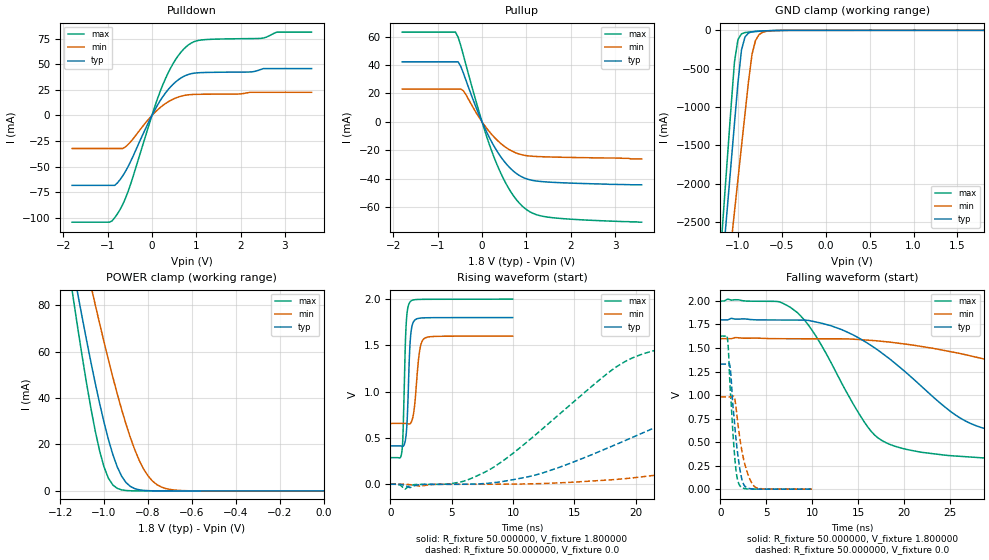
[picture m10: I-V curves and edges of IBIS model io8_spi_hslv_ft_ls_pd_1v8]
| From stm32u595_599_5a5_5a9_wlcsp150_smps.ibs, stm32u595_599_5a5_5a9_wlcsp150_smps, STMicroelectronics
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|   Model io8_spi_hslv_ft_ls_pd_1v8
[Model]  io8_spi_hslv_ft_ls_pd_1v8
Model_type I/O
Polarity   Non-Inverting
Enable   Active-Low
Vinl =   0.540000V
Vinh =   1.260000V
Vmeas =  0.900000V
Cref =   50.000000pF
Rref =   100.000000M
Vref =   0.0V
C_comp   3.338700pF   3.332500pF   3.379000pF
[Temperature Range]   25.000000   0.140000k   -40.000000
[Pullup Reference]   1.800000V   1.600000V   2.000000V
[Pulldown Reference]   0.0V   0.0V   0.0V
[POWER Clamp Reference]   1.800000V   1.600000V   2.000000V
[GND Clamp Reference]   0.0V   0.0V   0.0V
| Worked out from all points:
|   slope of the pulldown table from 0 to 0.27 V, typ, clamps not added: 13.6 ohm
|   slope of the pullup table from 0 to 0.27 V, typ, clamps not added: 15.9 ohm
|   GND clamp passes 1 mA (typ) near -0.50 V on its own axis
|   POWER clamp passes 1 mA (typ) near -0.86 V on its own axis
|   rising waveform, R_fixture 50.000000, V_fixture 1.800000: 20-80 % time 238ps typ, 381ps min, 212ps max; typ from 0.414 V to 1.8 V
|   rising waveform, R_fixture 50.000000, V_fixture 0.0: 20-80 % time 15.2ns typ, 31.7ns min, 8.92ns max; typ from 0 V to 1.33 V
|   falling waveform, R_fixture 50.000000, V_fixture 1.800000: 20-80 % time 10.9ns typ, 26.5ns min, 6.1ns max; typ from 1.8 V to 0.414 V
|   falling waveform, R_fixture 50.000000, V_fixture 0.0: 20-80 % time 792ps typ, 1.07ns min, 617ps max; typ from 1.33 V to 0 V
[Pulldown]
|Voltage   I(typ)   I(min)   I(max)
-1.8V     -68.38mA   -32.32mA   -104.4mA
-960mV    -68.38mA   -32.32mA   -104.4mA
-780mV    -66.07mA   -32.32mA   -96.42mA
-540mV    -50.22mA   -28.51mA   -74.66mA
0V        -10fA      -700fA     0A
240mV     18.04mA    9.598mA    29.41mA
480mV     30.68mA    16.02mA    50.95mA
780mV     39.47mA    19.98mA    67.56mA
1.14V     41.99mA    20.77mA    74.01mA
2.46V     45.09mA    22.69mA    75.44mA
2.82V     45.91mA    22.69mA    81.6mA
3.6V      45.91mA    22.69mA    81.6mA
[Pullup]
|Voltage   I(typ)   I(min)   I(max)
-1.8V     42.21mA    23.08mA    63.11mA
-600mV    42.21mA    23.08mA    63.11mA
-540mV    42.21mA    23.08mA    59.57mA
-420mV    34.21mA    21.83mA    46.75mA
0V        0A         0A         0A
300mV     -18.63mA   -11.6mA    -27.18mA
600mV     -31.41mA   -19.24mA   -46.67mA
780mV     -36.41mA   -22mA      -54.89mA
960mV     -39.54mA   -23.51mA   -60.64mA
1.2V      -41.44mA   -24.28mA   -64.93mA
1.56V     -42.42mA   -24.69mA   -67.24mA
3.6V      -44.2mA    -26mA      -70.5mA
[GND_clamp]
|Voltage   I(typ)   I(min)   I(max)
-1.8V     -9.908A    -9.683A    -9.994A
-1.2V     -3.383A    -4.084A    -2.934A
-1.16V    -2.841A    -3.655A    -2.294A
-1.12V    -2.299A    -3.226A    -1.656A
-1.04V    -1.218A    -2.369A    -414.2mA
-1V       -684.7mA   -1.941A    -119.2mA
-960mV    -257.2mA   -1.514A    -45.67mA
-920mV    -87.04mA   -1.089A    -28.94mA
-840mV    -19.36mA   -312.8mA   -18.98mA
-800mV    -13.56mA   -132.4mA   -15.51mA
-720mV    -8.053mA   -25.67mA   -9.504mA
1.8V      45.71uA    33.32uA    56.11uA
[POWER_clamp]
|Voltage   I(typ)   I(min)   I(max)
-1.8V     470.8mA    433.7mA    554.6mA
-1.14V    95.25mA    122.7mA    82.82mA
-1.12V    84.97mA    114mA      70.27mA
-1.06V    55.51mA    88.42mA    35.67mA
-1.04V    46.34mA    80.15mA    25.76mA
-1V       29.51mA    64.13mA    10.3mA
-940mV    10.39mA    41.86mA    1.109mA
-900mV    3.624mA    28.77mA    182.8uA
-840mV    490.7uA    13.24mA    11.35uA
-800mV    116.8uA    6.532mA    1.77uA
-740mV    13.2uA     1.724mA    109.3nA
0V        0A         18.75nA    0A
[Ramp]
| variable   typ   min   max
dV/dt_r  0.79740/15.22129n   0.58772/31.69284n   0.97632/8.91131n
dV/dt_f  0.83143/10.92816n   0.56537/26.52287n   1.02743/6.08253n
R_load = 50.000000
[Rising Waveform]
R_fixture= 50.000000
V_fixture= 1.800000
V_fixture_min= 1.600000
V_fixture_max= 2.000000
|time   V(typ)   V(min)   V(max)
0s        413.8mV    656.5mV    287.1mV
940.9ps   411.3mV    656.6mV    348mV
1.041ns   410.7mV    656.6mV    560.4mV
1.281ns   522.4mV    656.1mV    1.694V
1.401ns   766mV      654.2mV    1.883V
1.602ns   1.498V     653.4mV    1.967V
1.882ns   1.752V     752.7mV    1.99V
2.382ns   1.793V     1.432V     1.996V
2.763ns   1.797V     1.573V     1.997V
9.97ns    1.8V       1.599V     2V
[Rising Waveform]
R_fixture= 50.000000
V_fixture= 0.0
V_fixture_min= 0.0
V_fixture_max= 0.0
|time   V(typ)   V(min)   V(max)
0s        1.796nV    144.1nV    1.167nV
6.006ns   174.7uV    -417uV     33.66mV
11.61ns   92.14mV    5.044mV    508.6mV
19.62ns   499.4mV    66.91mV    1.357V
28.43ns   973.3mV    231.9mV    1.566V
34.43ns   1.162V     360.7mV    1.6V
42.44ns   1.255V     527.1mV    1.619V
59.66ns   1.313V     797.6mV    1.627V
77.28ns   1.325V     912.2mV    1.627V
199.4ns   1.329V     979.7mV    1.627V
[Falling Waveform]
R_fixture= 50.000000
V_fixture= 1.800000
V_fixture_min= 1.600000
V_fixture_max= 2.000000
|time   V(typ)   V(min)   V(max)
0s        1.8V       1.599V     2V
7.608ns   1.798V     1.598V     1.933V
10.01ns   1.785V     1.598V     1.684V
16.82ns   1.5V       1.578V     572.5mV
24.82ns   843mV      1.466V     357.4mV
28.43ns   653.8mV    1.389V     333.4mV
34.83ns   536.1mV    1.224V     310.5mV
48.45ns   458.9mV    910.5mV    293.6mV
64.06ns   430.4mV    771.9mV    288.6mV
199.4ns   413.8mV    656.5mV    287.1mV
[Falling Waveform]
R_fixture= 50.000000
V_fixture= 0.0
V_fixture_min= 0.0
V_fixture_max= 0.0
|time   V(typ)   V(min)   V(max)
0s        1.329V     979.7mV    1.627V
760.8ps   1.329V     979.8mV    1.606V
880.9ps   1.334V     979.9mV    1.465V
1.081ns   1.279V     979.7mV    1.039V
1.542ns   700.9mV    969.4mV    361.6mV
1.782ns   457mV      799.4mV    143.5mV
2.082ns   236.2mV    564.1mV    42.59mV
2.603ns   38.81mV    287.6mV    6.523mV
3.764ns   1.375mV    23.55mV    372.1uV
9.97ns    1.796nV    144.1nV    1.167nV
